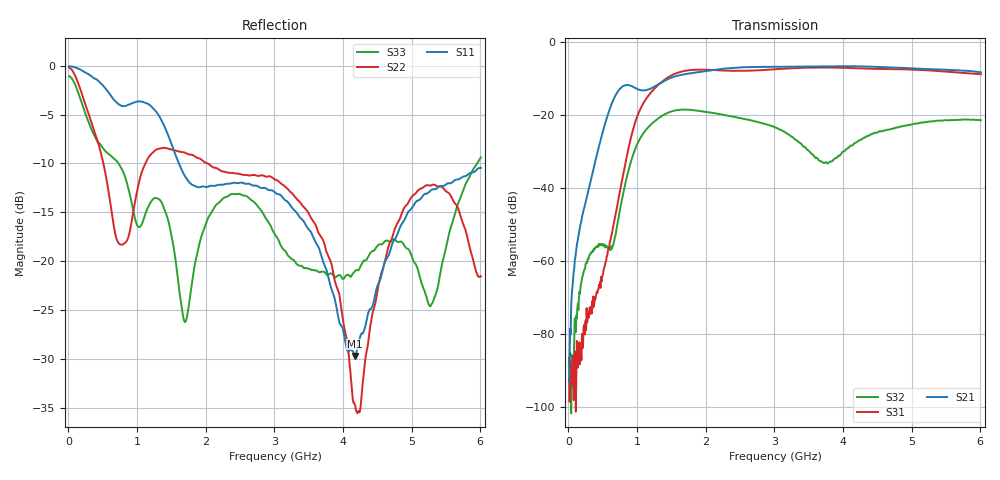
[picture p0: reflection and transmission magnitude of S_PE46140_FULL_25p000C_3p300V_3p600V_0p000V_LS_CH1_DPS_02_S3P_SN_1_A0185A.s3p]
! Device ID: PE46140_FULL
! File Path: z:\PE46140\MajorStates\25p000C\3p300\LS_CH1_DPS_02\PE46140_FULL_25p000C_3p300V_3p600V_0p000V_LS_CH1_DPS_02_S3P_SN_1_A0185A.s3p
! Serial: 1
! Lot: A0185A
! Temp: 25.000C
! VDD: 3.300
! VSS: 0.000
! Control_Hi: 3.600
! Control_Lo: 0.000
! Logic State: LS_CH1_DPS_02
! Port 1: RFIN
! Port 2: RFOUT1
! Port 3: RFOUT2
! ThroughPath:1-2
! IDD: 0.0003111281
! ISS: -1.221e-007
! Comment:
#  Hz  S  RI  R  50
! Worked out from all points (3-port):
!   801 points, 10 MHz to 6.01 GHz, reference 50 ohm
!   strongest paths, dB at 10 MHz, 1.51 GHz, 3.01 GHz, 4.51 GHz, 6.01 GHz:
!     S21: -92.9, -9.7, -6.8, -6.9, -8.3
!     S31: -86.5, -9.1, -7.5, -7.4, -8.9
!     S32: -88.3, -19.0, -23.4, -24.7, -21.4
!   lowest |S11| = -29.7 dB at 4.173 GHz (marker M1), VSWR 1.07, Z = 47 + j1.14 ohm
!   |S11| at or under -10 dB: 1.61 GHz to end of sweep
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1e7  0.9922 -0.0708  -3.9e-06 2.63e-05  -1.58e-05 -8.23e-06
     -1.32e-05 1.84e-05  0.9749 -0.0928  -7.02e-05 1.96e-05
     -4.1e-05 2.4e-05  -1.22e-05 3.64e-05  0.881 -0.0832
3.1e8  -0.2431 -0.862  -0.0106 0.00267  -7.33e-05 0.000183
       -0.0106 0.00266  -0.385 -0.3859  -0.000433 0.00105
       -0.000118 0.000199  -0.000497 0.0011  -0.3585 -0.3432
7.375e8  -0.6286 -0.0796  0.0457 0.2154  0.00768 -0.000204
         0.0456 0.2156  -0.1026 0.0673  -0.000729 0.00427
         0.00781 -0.000139  -0.000754 0.00419  0.0113 0.3126
1.36e9  -0.3305 0.4037  0.2342 -0.1525  -0.2042 0.1963
        0.2347 -0.1523  0.0126 0.3783  -0.0436 0.0864
        -0.2046 0.1963  -0.0436 0.0863  0.1918 -0.0526
1.6975e9  -0.1314 0.2378  0.0471 -0.3583  0.2744 0.2932
          0.047 -0.3586  0.2434 0.2636  0.1183 0.00045
          0.2745 0.2936  0.1184 0.00062  -0.0485 -0.00413
1.945e9  -0.1354 0.1987  -0.1679 -0.3541  0.4155 -0.032
         -0.1679 -0.3541  0.2918 0.1522  0.0371 -0.106
         0.4159 -0.0319  0.0373 -0.1058  0.0391 0.1307
3.01e9  0.0107 0.2242  -0.1731 0.4221  -0.3662 -0.2099
        -0.1741 0.4219  0.2244 -0.1343  0.0419 0.0529
        -0.3667 -0.2103  0.0421 0.0528  0.1271 -0.0501
4.1725e9  -0.0303 0.0121  0.4367 -0.1589  0.1101 0.4238
          0.4367 -0.1583  0.0126 -0.0134  0.0171 0.0376
          0.1102 0.4231  0.0172 0.0375  0.086 -0.0204
5.02e9  -0.1343 -0.134  -0.1955 -0.3868  0.4044 -0.1026
        -0.1951 -0.3874  0.2123 0.0409  -0.0426 -0.0616
        0.4043 -0.1029  -0.0426 -0.0614  0.0788 -0.0645
6.01e9  -0.2477 -0.169  -0.2132 0.3177  -0.164 -0.3205
        -0.2137 0.3179  0.0836 0.00272  0.0368 0.0763
        -0.165 -0.321  0.0375 0.0761  0.3168 0.1212
